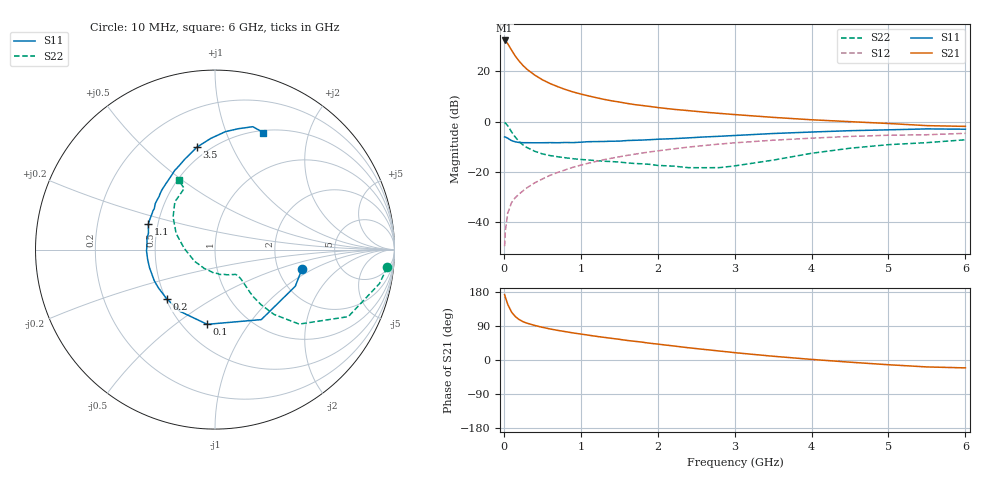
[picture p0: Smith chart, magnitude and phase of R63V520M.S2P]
! SIEMENS Small Signal Semiconductors
! BFR193
! Si NPN RF Bipolar Junction Transistor in SOT23
! VCE = 3.5 V  IC = 20 mA
! Common Emitter S-Parameters:  May  1996
# GHz  S  MA  R  50
!  f  S11  S21  S12  S22
! GHz  MAG  ANG  MAG  ANG  MAG  ANG  MAG  ANG
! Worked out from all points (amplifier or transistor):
!   36 points, 10 MHz to 6 GHz, reference 50 ohm
!   highest |S21| = 32.3 dB at 10 MHz (marker M1)
!   |S21| within 3 dB of that: start of sweep to 83.77 MHz
!   unconditionally stable (mu >= 1): 574.5 MHz to 1.93 GHz
!   at 250 MHz: K = 0.83, MSG = 24.9 dB, |S12| = -27.6 dB
!   at 1.4 GHz: K = 1.03, MAG = 10.5 dB, |S12| = -14.6 dB
!   at 6 GHz: K = 0.94, MSG = 1.4 dB, |S12| = -4.7 dB
!   lowest NFmin = 1.40 dB at 450 MHz
!   S11 on the Smith chart (normalised r, x): 10 MHz: 2.71, -0.79; 100 MHz: 0.65, -0.66; 200 MHz: 0.51, -0.32; 1.1 GHz: 0.44, +0.15; 3.5 GHz: 0.43, +0.74; 6 GHz: 0.52, +1.36
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0.01  0.4966 -12.7  41.42 172.6  0.0033 87.9  0.9644 -5.9
0.02  0.4918 -24.5  40.29 165.4  0.0067 80.5  0.9356 -11.7
0.05  0.4677 -56.5  35.84 147.1  0.0149 71.9  0.8312 -26.7
0.1  0.4186 -96.0  26.63 126.6  0.0243 64.1  0.6265 -41.5
0.15  0.3955 -119.5  20.1 114.3  0.0307 62.0  0.4881 -47.7
0.2  0.3839 -134.6  15.97 106.7  0.0362 63.1  0.4003 -50.1
0.25  0.3806 -145.7  13.09 101.0  0.0419 64.4  0.3412 -50.9
0.3  0.3803 -152.8  11.07 97.2  0.048 65.6  0.3054 -50.7
0.4  0.3786 -164.6  8.493 91.3  0.0601 67.2  0.2572 -49.6
0.5  0.3794 -172.4  6.837 86.3  0.0719 68.5  0.2278 -48.8
0.6  0.3816 -179.0  5.744 82.0  0.085 68.8  0.2107 -48.5
0.8  0.384 171.1  4.365 74.9  0.1096 68.1  0.1903 -49.4
0.9  0.3819 166.1  3.902 71.5  0.1233 67.8  0.1825 -49.8
1.1  0.3983 158.7  3.256 65.5  0.1485 66.2  0.1723 -54.0
1.3  0.4023 151.8  2.783 59.8  0.1745 64.2  0.1625 -58.0
1.6  0.4201 142.3  2.31 51.7  0.2118 60.6  0.1508 -67.3
2.2  0.4579 126.7  1.764 37.2  0.2859 52.8  0.13 -93.7
2.8  0.5101 112.7  1.461 23.8  0.3567 44.1  0.1211 -135.8
3.5  0.5796 100.0  1.216 9.9  0.4261 33.2  0.171 178.0
4.5  0.6599 84.9  0.999 -5.8  0.5071 18.9  0.2952 142.3
5.5  0.7163 72.9  0.832 -18.3  0.5477 4.6  0.3815 116.7
6  0.7058 67.5  0.804 -20.8  0.5845 0.3  0.4349 117.7
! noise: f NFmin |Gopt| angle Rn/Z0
0.45  1.4  0.3  160  0.1
0.9  1.45  0.34  172  0.11
1.8  2.2  0.56  -148  0.2
